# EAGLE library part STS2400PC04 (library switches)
SWITCH SLIDE 4POS VERT BLACK T/H
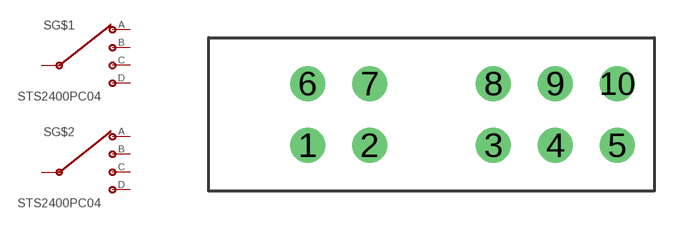
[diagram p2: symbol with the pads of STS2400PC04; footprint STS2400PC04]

Designator prefix S; gates G$1=SP4T G$2=SP4T

## STS2400PC04 (DIGIKEY: 450-1619-ND)  [STS2400PC04]
1  G$1:A
2  G$1:B
3  G$1:INPUT
4  G$1:C
5  G$1:D
6  G$2:A
7  G$2:B
8  G$2:INPUT
9  G$2:C
10  G$2:D

## Footprint STS2400PC04 (pad centres in mm)
drill 0.9: 1 -5,-1.245; 2 -2.5,-1.245; 3 2.5,-1.245; 4 5,-1.245; 5 7.5,-1.245; 6 -5,1.245; 7 -2.5,1.245; 8 2.5,1.245; 9 5,1.245; 10 7.5,1.245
